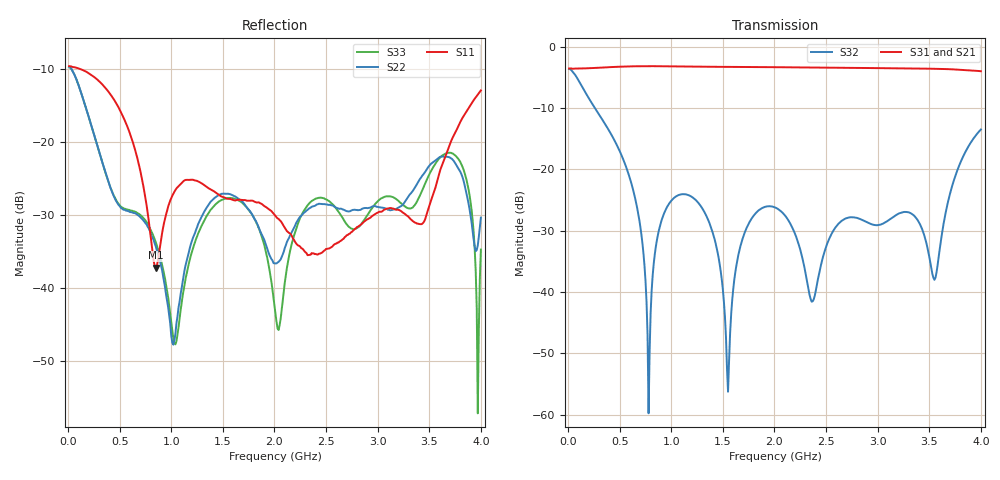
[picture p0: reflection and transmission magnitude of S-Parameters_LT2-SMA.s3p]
! MTS Systemtechnik GmbH
! S-Parameters
! Model: LT2-544P-4G
! Rohde & Schwarz ZVB8 2Ports - Version 3.20 - 1145.1010k08 SN: 100119
! Converted & adapted with MATLAB
!		|  MTS  |
!		|  |--o OUT 2 (Port 3)
! C (Port 1) o--| LT2-544P-4G |
!		|  |--o OUT 1 (Port 2)
! S3P File: Measurements:
! <S11,S12,S13>,
! <S21,S22,S23>,
! <S31,S32,S33>:
# HZ  S  DB  R  50.00
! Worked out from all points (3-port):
!   400 points, 10 MHz to 4 GHz, reference 50 ohm
!   strongest paths, dB at 10 MHz, 1.01 GHz, 2.01 GHz, 3.01 GHz, 4 GHz:
!     S31: -3.5, -3.2, -3.3, -3.5, -4.0
!     S21: -3.5, -3.2, -3.3, -3.5, -4.0
!     S32: -3.6, -24.9, -26.2, -29.0, -13.5
!   lowest |S11| = -37.2 dB at 850 MHz (marker M1), VSWR 1.03, Z = 50.3 + j1.36 ohm
!   |S11| at or under -10 dB: 128.7 MHz to end of sweep
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1e7  -9.55 177.6  -3.54 -2.7  -3.54 -2.6
     -3.53 -2.7  -9.65 171.9  -3.59 -5.5
     -3.54 -2.7  -3.59 -5.5  -9.64 172.0
6.5e8  -21.05 38.2  -3.17 -173.8  -3.16 -173.8
       -3.17 -173.8  -29.70 148.1  -24.72 162.5
       -3.17 -173.8  -24.72 162.6  -29.50 150.3
7.8e8  -30.56 27.8  -3.15 150.7  -3.15 150.7
       -3.16 150.7  -31.74 97.2  -59.74 74.8
       -3.15 150.7  -59.77 74.4  -31.39 99.3
8.5e8  -37.17 78.0  -3.16 131.6  -3.15 131.6
       -3.16 131.6  -34.25 73.5  -32.63 -67.6
       -3.16 131.5  -32.63 -67.6  -33.67 76.0
1.34e9  -26.06 67.1  -3.24 -1.5  -3.24 -1.5
        -3.24 -1.5  -29.00 57.7  -27.57 161.8
        -3.24 -1.5  -27.58 161.9  -30.15 64.9
1.55e9  -27.72 55.1  -3.27 -58.6  -3.27 -58.6
        -3.26 -58.6  -27.02 0.3  -56.42 -156.0
        -3.27 -58.6  -56.25 -157.2  -27.60 4.0
2.01e9  -30.07 12.0  -3.32 175.9  -3.32 175.9
        -3.32 175.9  -36.57 -57.0  -26.23 162.7
        -3.32 175.9  -26.23 162.6  -43.52 -85.7
3.73e9  -19.24 141.2  -3.66 57.1  -3.67 57.1
        -3.66 57.0  -22.42 -145.6  -22.21 132.6
        -3.67 57.1  -22.22 132.6  -21.55 -144.9
3.97e9  -13.45 88.8  -3.91 -11.7  -3.92 -11.7
        -3.91 -11.7  -34.11 -92.1  -14.04 70.9
        -3.93 -11.7  -14.04 70.9  -57.11 130.9
4e9  -12.87 81.9  -3.95 -20.4  -3.97 -20.3
     -3.95 -20.4  -30.30 -69.4  -13.48 62.7
     -3.97 -20.3  -13.48 62.6  -34.68 -30.0
